FUNCTION "ABILIT_ACP" : VOID
TITLE =ABILITAZIONE E GESTIONE ERRORI ACP600
VERSION : 0.1

BEGIN
NETWORK
TITLE =LETTURA INGRESSO STATO ACP 600
//BIT DELLA CONTROL WORD:
//DBX255.0 = BIT 0 READY TO OPERATE
//DBX255.1 = BIT 1 OFF1 INACTIVE
//DBX255.2 = BIT 2 OFF2 INACTIVE
//DBX254.2 = BIT 10 REMOTE COMMAND
//
//BIT DELLA STATUS WORD:
//DBX243.0 = BIT 0 READY TO SWITCH ON
//DBX243.1 = BIT 1 READY TO OPERATE
//DBX243.2 = BIT 2 OPERATION ENABLED
//DBX243.3 = BIT 3 FAULT
//DBX243.6 = BIT 6 SWITCH-ON INHIBITED
//DBX242.1 = BIT 9 REMOTE COMMAND
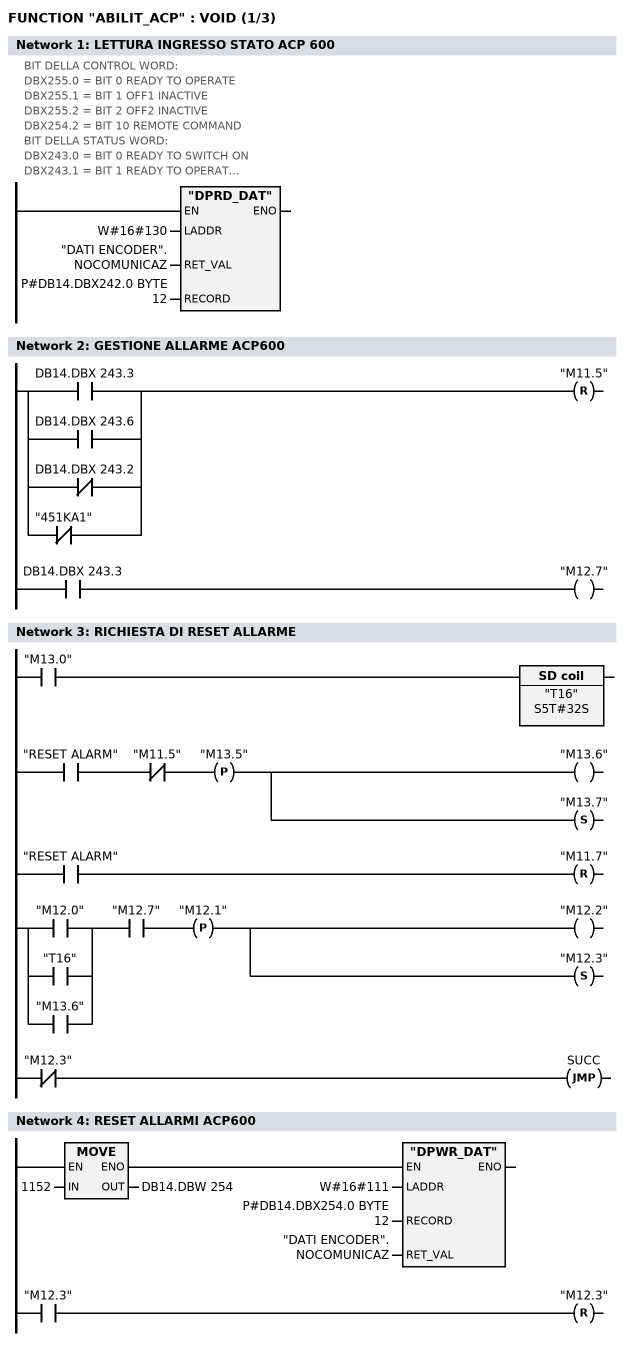
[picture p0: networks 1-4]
      CALL "DPRD_DAT" (
           LADDR                    := W#16#130,
           RET_VAL                  := "DATI ENCODER".NOCOMUNICAZ,
           RECORD                   := P#DB14.DBX242.0 BYTE 12);

NETWORK
TITLE =GESTIONE ALLARME ACP600

      U     DB14.DBX  243.3;
      O     DB14.DBX  243.6;
      ON    DB14.DBX  243.2;
      ON    "451KA1";
      R     "M11.5";

      U     DB14.DBX  243.3;
      =     "M12.7";
NETWORK
TITLE =RICHIESTA DI RESET ALLARME

      U     "M13.0";
      L     S5T#32S;
      SE    "T16";

      U     "RESET ALARM";
      UN    "M11.5";
      FP    "M13.5";
      =     "M13.6";
      S     "M13.7";

      U     "RESET ALARM";
      R     "M11.7";

      U     "M12.0";
      O     "T16";
      O     "M13.6";
      U     "M12.7";
      FP    "M12.1";
      =     "M12.2";
      S     "M12.3";

      UN    "M12.3";
      SPB   SUCC;

NETWORK
TITLE =RESET ALLARMI ACP600

      L     1152;
      T     DB14.DBW  254;

      CALL "DPWR_DAT" (
           LADDR                    := W#16#111,
           RECORD                   := P#DB14.DBX254.0 BYTE 12,
           RET_VAL                  := "DATI ENCODER".NOCOMUNICAZ);

      U     "M12.3";
      R     "M12.3";

NETWORK
TITLE =RICHIESTA DI ABILITAZIONE
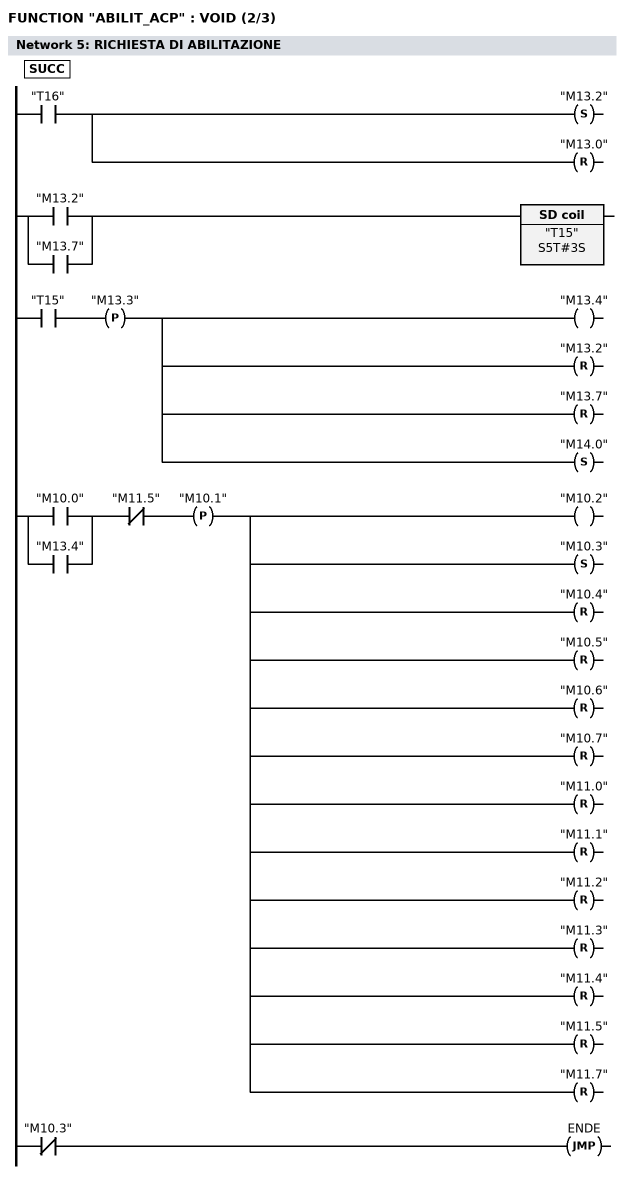
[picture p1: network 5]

SUCC: U     "T16";
      S     "M13.2";
      R     "M13.0";

      U     "M13.2";
      O     "M13.7";
      L     S5T#3S;
      SE    "T15";

      U     "T15";
      FP    "M13.3";
      =     "M13.4";
      R     "M13.2";
      R     "M13.7";
      S     "M14.0";

      U     "M10.0";
      O     "M13.4";
      UN    "M11.5";
      FP    "M10.1";
      =     "M10.2";
      S     "M10.3";
      R     "M10.4";
      R     "M10.5";
      R     "M10.6";
      R     "M10.7";
      R     "M11.0";
      R     "M11.1";
      R     "M11.2";
      R     "M11.3";
      R     "M11.4";
      R     "M11.5";
      R     "M11.7";

      UN    "M10.3";
      SPB   ENDE;

NETWORK
TITLE =GESTIONE PASSI INTERMEDI
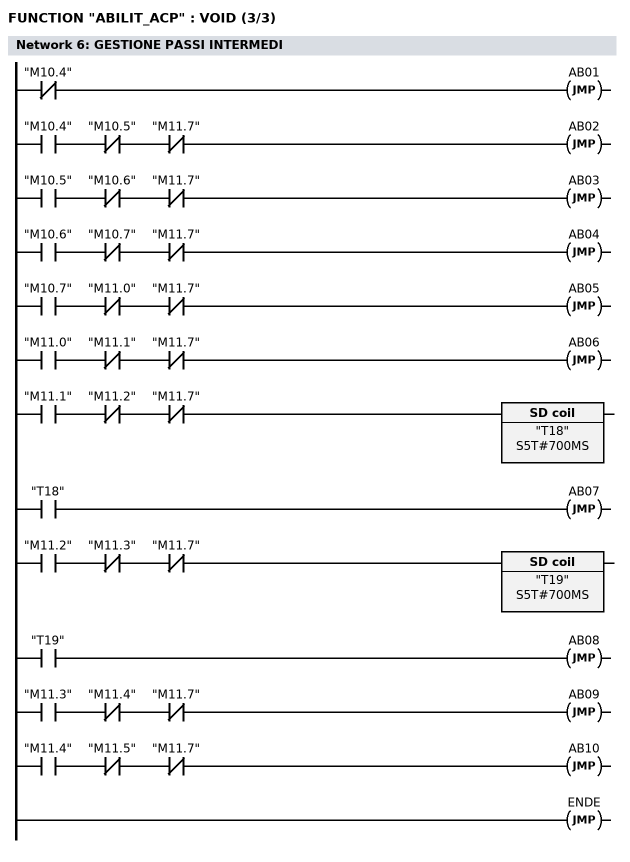
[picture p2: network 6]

      UN    "M10.4";
      SPB   AB01;

      U     "M10.4";
      UN    "M10.5";
      UN    "M11.7";
      SPB   AB02;

      U     "M10.5";
      UN    "M10.6";
      UN    "M11.7";
      SPB   AB03;

      U     "M10.6";
      UN    "M10.7";
      UN    "M11.7";
      SPB   AB04;

      U     "M10.7";
      UN    "M11.0";
      UN    "M11.7";
      SPB   AB05;

      U     "M11.0";
      UN    "M11.1";
      UN    "M11.7";
      SPB   AB06;

      U     "M11.1";
      UN    "M11.2";
      UN    "M11.7";
      L     S5T#700MS;
      SE    "T18";
      U     "T18";
      SPB   AB07;

      U     "M11.2";
      UN    "M11.3";
      UN    "M11.7";
      L     S5T#700MS;
      SE    "T19";
      U     "T19";
      SPB   AB08;

      U     "M11.3";
      UN    "M11.4";
      UN    "M11.7";
      SPB   AB09;

      U     "M11.4";
      UN    "M11.5";
      UN    "M11.7";
      SPB   AB10;
      SPA   ENDE;

NETWORK
TITLE =PASSO 1: AZZERO LA CW

AB01: L     1024;
      T     DB14.DBW  254;

      CALL "DPWR_DAT" (
           LADDR                    := W#16#111,
           RECORD                   := P#DB14.DBX254.0 BYTE 12,
           RET_VAL                  := "DATI ENCODER".NOCOMUNICAZ);

      U     "M10.3";
      S     "M10.4";
      SPA   ENDE;
NETWORK
TITLE =PASSO 2: ASPETTO CHE LA SW SIA RESETTATA
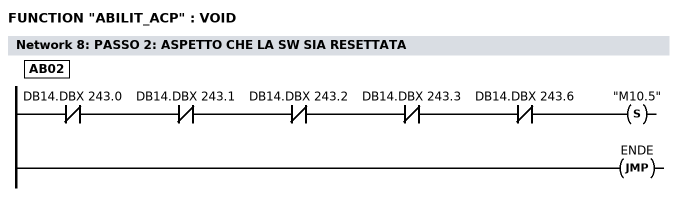
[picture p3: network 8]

AB02: UN    DB14.DBX  243.0;
      UN    DB14.DBX  243.1;
      UN    DB14.DBX  243.2;
      UN    DB14.DBX  243.3;
      UN    DB14.DBX  243.6;
      S     "M10.5";

      SPA   ENDE;
NETWORK
TITLE =PASSO 3: DISABILITO GLI OFF

AB03: L     1030;
      T     DB14.DBW  254;

      CALL "DPWR_DAT" (
           LADDR                    := W#16#111,
           RECORD                   := P#DB14.DBX254.0 BYTE 12,
           RET_VAL                  := "DATI ENCODER".NOCOMUNICAZ);

      U     "M10.3";
      S     "M10.6";

      SPA   ENDE;

NETWORK
TITLE =PASSO 4: ASPETTO CHE LA SW SIA IN READY TO SWITCH ON

AB04: U     DB14.DBX  243.0;
      S     "M10.7";

      SPA   ENDE;

NETWORK
TITLE =PASSO 5: DO IL READY TO OPERATE

AB05: L     1031;
      T     DB14.DBW  254;

      CALL "DPWR_DAT" (
           LADDR                    := W#16#111,
           RECORD                   := P#DB14.DBX254.0 BYTE 12,
           RET_VAL                  := "DATI ENCODER".NOCOMUNICAZ);

      U     "M10.3";
      S     "M11.0";

      SPA   ENDE;

NETWORK
TITLE =PASSO 6: ASPETTO CHE LA SW SIA IN READY TO OPERATE

AB06: U     DB14.DBX  243.1;
      S     "M11.1";

      SPA   ENDE;
NETWORK
TITLE =PASSO 7: DO IL RUN

AB07: L     1039;
      T     DB14.DBW  254;

      CALL "DPWR_DAT" (
           LADDR                    := W#16#111,
           RECORD                   := P#DB14.DBX254.0 BYTE 12,
           RET_VAL                  := "DATI ENCODER".NOCOMUNICAZ);

      U     "M10.3";
      S     "M11.2";
      SPA   ENDE;
NETWORK
TITLE =PASSO 8: DO IL POSITION ENABLED

AB08: L     1071;
      T     DB14.DBW  254;

      CALL "DPWR_DAT" (
           LADDR                    := W#16#111,
           RECORD                   := P#DB14.DBX254.0 BYTE 12,
           RET_VAL                  := "DATI ENCODER".NOCOMUNICAZ);

      U     "M10.3";
      S     "M11.3";
      SPA   ENDE;


NETWORK
TITLE =PASSO 8: ASPETTO CHE SIA IN OPERATION ENABLED
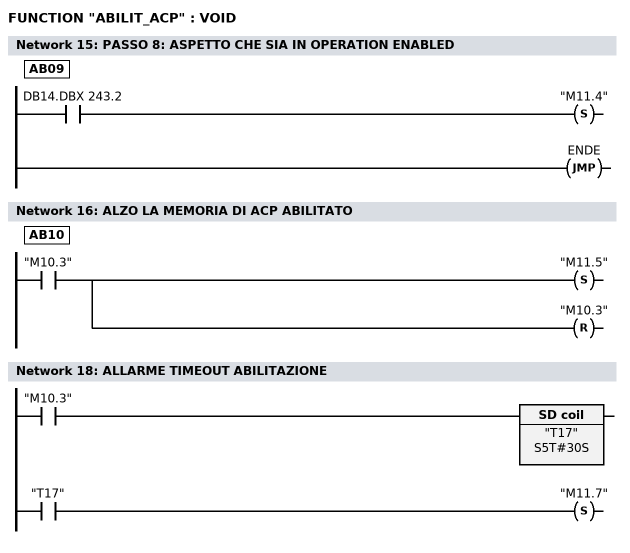
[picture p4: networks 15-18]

AB09: U     DB14.DBX  243.2;
      S     "M11.4";

      SPA   ENDE;

NETWORK
TITLE =ALZO LA MEMORIA DI ACP ABILITATO

AB10: U     "M10.3";
      S     "M11.5";
      R     "M10.3";

NETWORK
TITLE =

ENDE: NOP   0;

NETWORK
TITLE =ALLARME TIMEOUT ABILITAZIONE

      U     "M10.3";
      L     S5T#30S;
      SE    "T17";
      U     "T17";
      S     "M11.7";

END_FUNCTION

